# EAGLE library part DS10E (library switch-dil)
DIL/CODE SWITCH
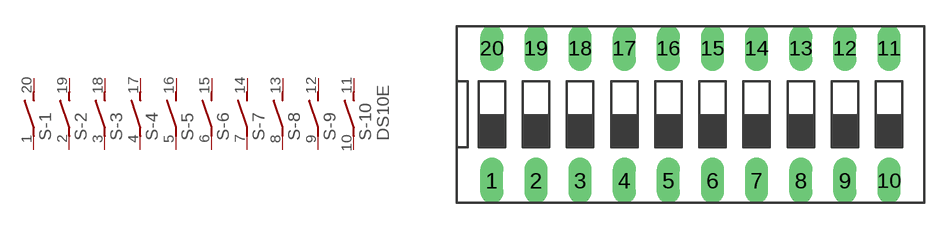
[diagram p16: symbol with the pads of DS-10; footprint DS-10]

Designator prefix S; gates -1=S -2=S -3=S -4=S -5=S -6=S -7=S -8=S -9=S -10=S+V

## DS10E (OC_FARNELL: unknown; OC_NEWARK: unknown)  [DS-10]
1  -1:1  pas
2  -2:1  pas
3  -3:1  pas
4  -4:1  pas
5  -5:1  pas
6  -6:1  pas
7  -7:1  pas
8  -8:1  pas
9  -9:1  pas
10  -10:1  pas
11  -10:2  pas
12  -9:2  pas
13  -8:2  pas
14  -7:2  pas
15  -6:2  pas
16  -5:2  pas
17  -4:2  pas
18  -3:2  pas
19  -2:2  pas
20  -1:2  pas

## Footprint DS-10 (pad centres in mm)
DIL/CODE SWITCH Mors distributor Buerklin, 17G566
drill 0.813 long: 1 -11.43,-3.81; 2 -8.89,-3.81; 3 -6.35,-3.81; 4 -3.81,-3.81; 5 -1.27,-3.81; 6 1.27,-3.81; 7 3.81,-3.81; 8 6.35,-3.81; 9 8.89,-3.81; 10 11.43,-3.81; 11 11.43,3.81; 12 8.89,3.81; 13 6.35,3.81; 14 3.81,3.81; 15 1.27,3.81; 16 -1.27,3.81; 17 -3.81,3.81; 18 -6.35,3.81; 19 -8.89,3.81; 20 -11.43,3.81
